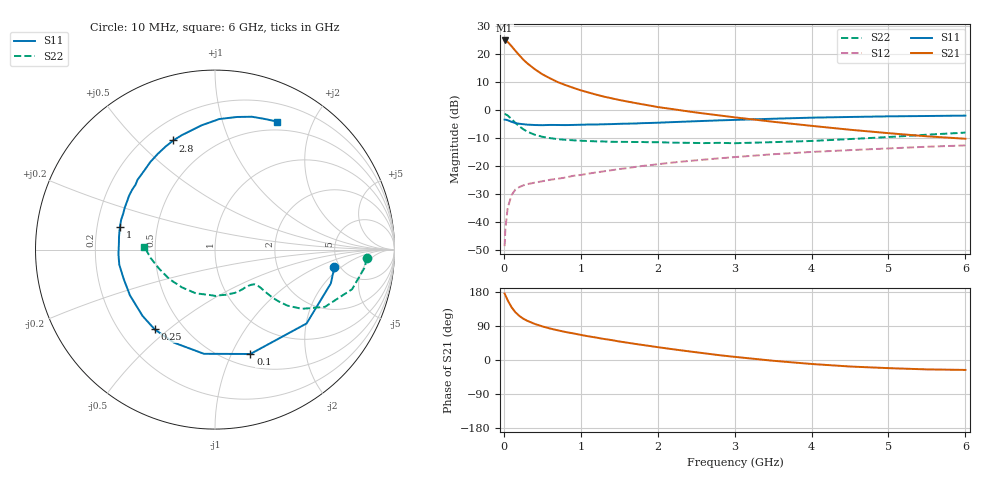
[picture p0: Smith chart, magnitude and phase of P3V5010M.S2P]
! SIEMENS Small Signal Semiconductors
! BFP181
! Si NPN RF Bipolar Junction Transistor in SOT143
! VCE = 0.5 V  IC = 10 mA
! Common Emitter S-Parameters:  March  1996
# GHz  S  MA  R  50
!  f  S11  S21  S12  S22
! GHz  MAG  ANG  MAG  ANG  MAG  ANG  MAG  ANG
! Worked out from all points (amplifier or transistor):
!   36 points, 10 MHz to 6 GHz, reference 50 ohm
!   highest |S21| = 24.8 dB at 10 MHz (marker M1)
!   |S21| within 3 dB of that: start of sweep to 129.3 MHz
!   unconditionally stable (mu >= 1): start of sweep to 13.04 MHz; 347.2 MHz to end of sweep
!   at 250 MHz: K = 0.77, MSG = 22.5 dB, |S12| = -27.0 dB
!   at 1.4 GHz: K = 2.27, MAG = 6.5 dB, |S12| = -21.5 dB
!   at 6 GHz: K = 2.29, MAG = -5.2 dB, |S12| = -12.7 dB
!   S11 on the Smith chart (normalised r, x): 10 MHz: 4.53, -1.58; 100 MHz: 0.63, -1.18; 250 MHz: 0.35, -0.45; 1 GHz: 0.30, +0.11; 2.8 GHz: 0.30, +0.64; 6 GHz: 0.40, +1.52
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0.01  0.6724 -8.2  17.39 175.5  0.0037 81.6  0.8457 -3.1
0.02  0.6723 -16.3  17.31 171.0  0.0075 75.7  0.8406 -6.7
0.05  0.6555 -38.9  16.37 157.5  0.0179 71.1  0.7951 -16.1
0.1  0.6141 -71.3  13.75 139.3  0.0301 55.3  0.6907 -27.5
0.15  0.5839 -96.1  11.38 126.0  0.0379 46.5  0.5857 -34.3
0.2  0.5665 -113.8  9.491 116.6  0.0419 41.6  0.5108 -37.7
0.25  0.5571 -127.1  7.995 109.3  0.0449 38.3  0.4549 -39.2
0.3  0.5473 -137.5  6.884 103.9  0.0472 36.4  0.4126 -39.9
0.4  0.5381 -151.7  5.36 95.3  0.0503 35.3  0.3611 -40.0
0.5  0.5344 -162.3  4.338 88.7  0.0533 34.6  0.3325 -39.9
0.6  0.5399 -171.1  3.67 83.1  0.0566 35.6  0.3139 -40.1
0.7  0.5386 -177.4  3.142 78.4  0.0592 36.6  0.3009 -40.6
0.8  0.5363 176.8  2.782 74.0  0.0621 37.4  0.2929 -41.3
1  0.5445 166.8  2.24 66.3  0.0691 39.1  0.2823 -43.9
1.1  0.5486 162.4  2.048 62.5  0.0731 39.8  0.2783 -45.4
1.5  0.5648 148.1  1.507 48.9  0.088 40.6  0.2694 -53.0
2.2  0.6066 126.5  1.031 28.3  0.1152 38.6  0.2603 -71.2
2.8  0.6512 110.9  0.799 12.7  0.1369 35.0  0.2584 -89.0
3.5  0.6963 96.2  0.615 -2.0  0.1619 29.8  0.266 -113.6
4.5  0.7489 80.6  0.443 -17.2  0.1917 20.8  0.3022 -146.8
5.5  0.7792 69.0  0.338 -24.8  0.2203 12.5  0.3612 -172.4
6  0.7927 64.1  0.306 -26.2  0.2327 7.8  0.394 177.6
